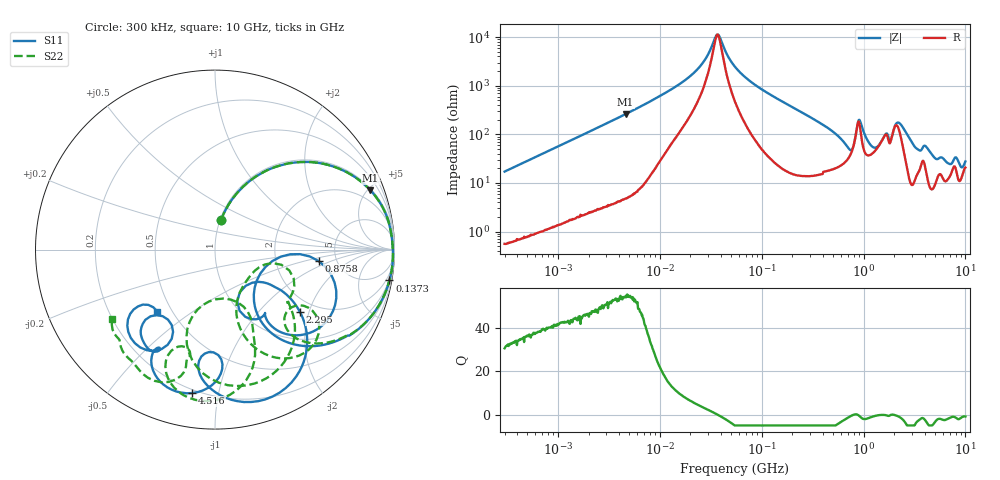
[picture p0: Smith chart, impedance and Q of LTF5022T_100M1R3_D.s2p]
! S-Parameter Data Generated by TDK Corporation
! Copyright(C) 2020 TDK Corporation.
! All Rights Reserved.
! TDK P/N: LTF5022T-100M1R3-D (Inductor)
! Property: L=10uH at 100kHz
! Size(LxWxT): 6.5x5x2.2mm
! Model Type: s2p (Touchstone File Format Version 1.0)
! Frequency: DC=Yes Start=0.3MHz Stop=10000MHz 802points Log-sweep
! Model Generated on Apr. 23, 2020
! Port Assignments:
!  1 ---@@@--- 2
! Applicable Conditions:
!  Temperature = 25 degC
!  DC Bias Current = 0 A
!  Small Signal Operation
! Terms and conditions regarding TDK Simulation Models
! (1)This simulation model is being provided solely for informational purposes. Please refer to the specifications of the products in terms of detailed characteristics of such products.
! (2)In no event shall TDK Corporation of any of its subsidiaries be liable for any loss or damage arising, directly or indirectly,
!  From any information contained in this simulation model, including, but not limited to loss or damages arising from any inaccuracies, omissions or errors in connection with such information.
! (3)Any and all copyrights on this simulation model are owned by TDK Corporation.
!  Duplication or redistribution of this simulation model without prior written permission from TDK Corporation is prohibited.
! (4)This simulation model is subject to any modification or change without any prior notice.
! (5)Neither TDK Corporation nor any of its subsidiaries shall make any warranty, express or implied,
!  Including but not limited to the correctness, implied warranties of merchantability and fitness for a particular purpose with respect to this simulation models.
! (6)The use of this simulation model shall be deemed to have consented to the terms and conditions hereof.
# Hz S MA R 50
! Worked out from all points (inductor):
!   801 points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, 300 kHz to 10 GHz, reference 50 ohm
!   read as 1/Y11, port 2 shorted: L = 9.09 uH near 318.3 kHz
!   highest Q = 54.4 at 4.611 MHz (marker M1), where L = 8.99 uH
!   self-resonance near 36.86 MHz
!   S11 on the Smith chart (normalised r, x): 300 kHz: 1.01, +0.34; 137.3 MHz: 1, -11; 875.8 MHz: 3.63, -0.69; 2.295 GHz: 1.64, -1.76; 4.516 GHz: 0.18, -0.84; 10 GHz: 0.42, -0.37
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300000  0.1688 78.5  0.9801 -9.7  0.9802 -9.7  0.1687 78.4
1713600  0.6847 45.5  0.7135 -43.2  0.7136 -43.2  0.6846 45.5
4611084  0.927 20.9  0.3584 -68.1  0.3584 -68.1  0.927 20.9
9671944  0.9782 9.6  0.1711 -78.1  0.1711 -78.1  0.9782 9.5
2.725275e7  0.9896 1.7  0.04419 -76.1  0.04419 -76.1  0.9896 1.7
4.625158e7  0.9918 -1.3  0.008268 -12.8  0.008265 -12.9  0.9918 -1.3
5.477226e7  0.9922 -2.3  0.01376 53.9  0.01376 53.9  0.9922 -2.3
1.372768e8  0.987 -10.0  0.1034 75.9  0.1034 75.8  0.9871 -10.0
3.126428e8  0.9361 -25.2  0.2713 59.5  0.2712 59.5  0.937 -24.9
7.400828e8  0.3862 -54.9  0.599 -3.7  0.5987 -3.7  0.5407 -44.2
8.758105e8  0.5806 -6.3  0.3187 -32.1  0.3185 -32.1  0.7247 -36.7
1.228555e9  0.5487 -53.0  0.576 -15.2  0.5752 -15.2  0.4273 -72.4
1.767019e9  0.4112 -65.7  0.4531 -65.9  0.4515 -65.9  0.3282 -13.2
2.294622e9  0.5895 -36.4  0.4738 -94.9  0.4725 -94.7  0.6084 -43.1
3.008786e9  0.8782 -74.1  0.08761 -93.2  0.08824 -93.7  0.693 -95.5
3.556288e9  0.6772 -97.7  0.228 -86.7  0.2226 -85.2  0.2769 -80.0
4.516006e9  0.8092 -99.0  0.1817 -148.6  0.1831 -148.2  0.7951 -81.5
4.924213e9  0.7955 -112.7  0.08955 -117.1  0.09077 -117.0  0.8384 -99.9
6.010849e9  0.6378 -118.9  0.2586 -148.8  0.2585 -148.5  0.5732 -105.1
7.316673e9  0.5518 -134.8  0.07235 164.9  0.06679 167.2  0.755 -106.7
8.658336e9  0.686 -127.4  0.1171 146.9  0.1215 147.5  0.7715 -130.0
1e10  0.4714 -133.0  0.02672 -179.1  0.03366 -178.3  0.6897 -146.1
